FUNCTION_BLOCK FB_AdsSend_A_To_B
VAR_INPUT
    xExecute       : BOOL;
    sRemoteNetId   : T_AmsNetId;
    nRemoteAdsPort : T_AmsPort := 851;
    sRemoteSymbol  : STRING(80);
    stData         : ST_A_To_B;
END_VAR
VAR_OUTPUT
    xBusy  : BOOL;
    xDone  : BOOL;
    xError : BOOL;
    nErrId : UDINT;
END_VAR
VAR
    fbTrig          : R_TRIG;
    fbGetHandle     : ADSRDWRT;
    fbWriteValue    : ADSWRITE;
    fbReleaseHandle : ADSWRITE;

    eState          : E_AdsWriteState := E_AdsWriteState.Idle;
    stTxBuffer      : ST_A_To_B;
    nSymbolHandle   : UDINT;

    xGetHandle      : BOOL;
    xWriteValue     : BOOL;
    xReleaseHandle  : BOOL;

    bGetBusy        : BOOL;
    bGetErr         : BOOL;
    nGetErrId       : UDINT;

    bWriteBusy      : BOOL;
    bWriteErr       : BOOL;
    nWriteErrId     : UDINT;

    bReleaseBusy    : BOOL;
    bReleaseErr     : BOOL;
    nReleaseErrId   : UDINT;
END_VAR

fbTrig(CLK := xExecute);

xDone := FALSE;
xError := FALSE;
nErrId := 0;

CASE eState OF
    E_AdsWriteState.Idle:
        xBusy := FALSE;
        xGetHandle := FALSE;
        xWriteValue := FALSE;
        xReleaseHandle := FALSE;

        IF fbTrig.Q THEN
            stTxBuffer := stData;
            xBusy := TRUE;
            eState := E_AdsWriteState.StartGetHandle;
        END_IF

    E_AdsWriteState.StartGetHandle:
        xBusy := TRUE;
        xGetHandle := TRUE;
        eState := E_AdsWriteState.WaitGetHandle;

    E_AdsWriteState.WaitGetHandle:
        xGetHandle := FALSE;
        xBusy := TRUE;

        IF NOT bGetBusy THEN
            IF bGetErr THEN
                xError := TRUE;
                nErrId := nGetErrId;
                eState := E_AdsWriteState.Idle;
            ELSE
                eState := E_AdsWriteState.StartWriteValue;
            END_IF
        END_IF

    E_AdsWriteState.StartWriteValue:
        xBusy := TRUE;
        xWriteValue := TRUE;
        eState := E_AdsWriteState.WaitWriteValue;

    E_AdsWriteState.WaitWriteValue:
        xWriteValue := FALSE;
        xBusy := TRUE;

        IF NOT bWriteBusy THEN
            IF bWriteErr THEN
                xError := TRUE;
                nErrId := nWriteErrId;
            ELSE
                xDone := TRUE;
            END_IF

            eState := E_AdsWriteState.StartReleaseHandle;
        END_IF

    E_AdsWriteState.StartReleaseHandle:
        xBusy := TRUE;
        xReleaseHandle := TRUE;
        eState := E_AdsWriteState.WaitReleaseHandle;

    E_AdsWriteState.WaitReleaseHandle:
        xReleaseHandle := FALSE;
        xBusy := TRUE;

        IF NOT bReleaseBusy THEN
            IF bReleaseErr AND NOT xError THEN
                xError := TRUE;
                nErrId := nReleaseErrId;
            END_IF

            eState := E_AdsWriteState.Idle;
        END_IF
END_CASE

fbGetHandle(
    NETID    := sRemoteNetId,
    PORT     := nRemoteAdsPort,
    IDXGRP   := 16#F003,
    IDXOFFS  := 0,
    WRITELEN := TO_UDINT(LEN(sRemoteSymbol) + 1),
    READLEN  := SIZEOF(nSymbolHandle),
    SRCADDR  := ADR(sRemoteSymbol),
    DESTADDR := ADR(nSymbolHandle),
    WRTRD    := xGetHandle,
    TMOUT    := T#5s,
    BUSY     => bGetBusy,
    ERR      => bGetErr,
    ERRID    => nGetErrId
);

fbWriteValue(
    NETID   := sRemoteNetId,
    PORT    := nRemoteAdsPort,
    IDXGRP  := 16#F005,
    IDXOFFS := nSymbolHandle,
    LEN     := SIZEOF(stTxBuffer),
    SRCADDR := ADR(stTxBuffer),
    WRITE   := xWriteValue,
    TMOUT   := T#5s,
    BUSY    => bWriteBusy,
    ERR     => bWriteErr,
    ERRID   => nWriteErrId
);

fbReleaseHandle(
    NETID   := sRemoteNetId,
    PORT    := nRemoteAdsPort,
    IDXGRP  := 16#F006,
    IDXOFFS := 0,
    LEN     := SIZEOF(nSymbolHandle),
    SRCADDR := ADR(nSymbolHandle),
    WRITE   := xReleaseHandle,
    TMOUT   := T#5s,
    BUSY    => bReleaseBusy,
    ERR     => bReleaseErr,
    ERRID   => nReleaseErrId
);

END_FUNCTION_BLOCK
